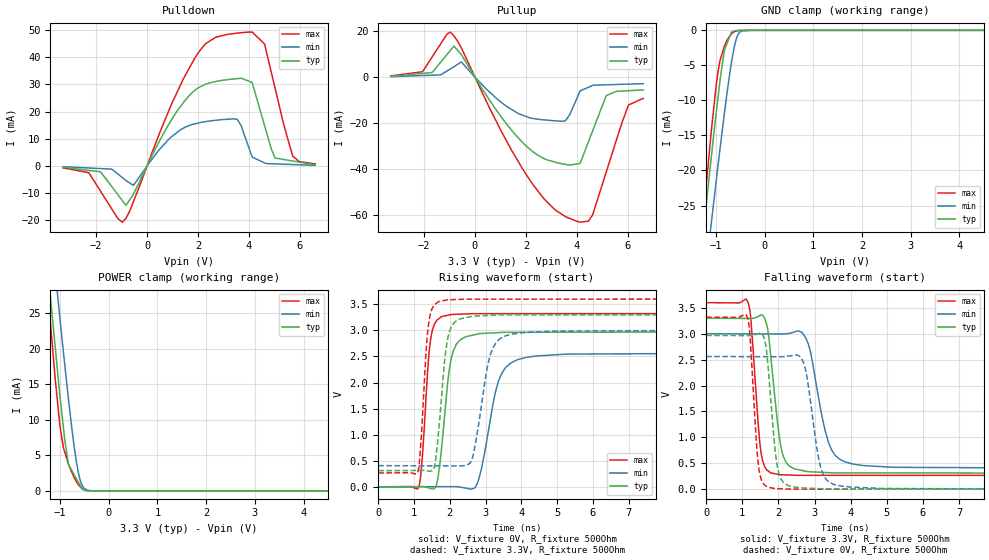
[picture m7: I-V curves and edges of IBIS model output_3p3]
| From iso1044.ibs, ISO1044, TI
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|   output_3p3 Model
[Model]   output_3p3
Model_type   3-state
Polarity   Inverting
Vmeas = 1.65
Vref = 0
Cref = 2pF
Rref = 100000
|   typ   min   max
C_comp   1.207pF   1.163pF   1.293pF
|C_comp_pullup   1.116pF   1.152pF   1.147pF
|C_comp_pulldown   1.051pF   1.086pF   1.093pF
|  Where Nom  PVT is Nominal Process, 3.3V,   27C
|   Fast PVT is Strong Process,  3.0V,   -40C
|   Slow PVT is Weak Process,   3.6V,   150C
[Voltage Range]   3.3   3   3.6
|Junction Temperature
[Temperature Range]   27   150   -40
[Pullup Reference]   3.3   3   3.6
[Pulldown Reference]   0   0   0
[Power Clamp Reference]   3.3   3   3.6
[GND Clamp Reference]   0   0   0
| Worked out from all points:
|   slope of the pulldown table from 0 to 0.495 V, typ, clamps not added: 53.2 ohm
|   slope of the pullup table from 0 to 0.495 V, typ, clamps not added: 56.8 ohm
|   GND clamp passes 1 mA (typ) near -0.72 V on its own axis
|   POWER clamp passes 1 mA (typ) near -0.60 V on its own axis
|   falling waveform, V_fixture 3.3V, R_fixture 500Ohm: 20-80 % time 280ps typ, 442ps min, 206ps max; typ from 3.3 V to 0.31 V
|   rising waveform, V_fixture 0V, R_fixture 500Ohm: 20-80 % time 270ps typ, 441ps min, 192ps max; typ from 0 V to 2.97 V
|   rising waveform, V_fixture 3.3V, R_fixture 500Ohm: 20-80 % time 241ps typ, 373ps min, 177ps max; typ from 0.31 V to 3.3 V
|   falling waveform, V_fixture 0V, R_fixture 500Ohm: 20-80 % time 224ps typ, 322ps min, 175ps max; typ from 2.97 V to 0 V
[Pulldown]
|   Voltage   I(typ)   I(min)   I(max)
-3.3V     -457.3uA   -258uA     -669.3uA
-2.283V   -1.618mA   -733.3uA   -2.463mA
-965.9mV  -12.74mA   -4.286mA   -20.68mA
-542.2mV  -10.56mA   -7.1mA     -13.32mA
871.8mV   15.6mA     10.03mA    20.74mA
2.011V    28.78mA    15.81mA    41.7mA
3.548V    32.16mA    17.07mA    48.91mA
3.983V    31.25mA    7.027mA    49.28mA
4.61V     14.86mA    1.146mA    44.88mA
5.023V    2.931mA    776.7uA    28.62mA
5.712V    1.841mA    543.7uA    3.669mA
6.6V      438.1uA    243.9uA    769.3uA
[GND Clamp]
|   Voltage   I(typ)   I(min)   I(max)
-3.3V     -171.9mA   -168.4mA   -191.9mA
-1.407V   -38.97mA   -46.94mA   -38.27mA
-1.251V   -28.45mA   -37.22mA   -26.03mA
-1.092V   -18mA      -27.4mA    -14.24mA
-951.9mV  -9.366mA   -19.05mA   -5.726mA
-825mV    -2.851mA   -11.84mA   -2.254mA
-683.5mV  -286.5uA   -4.778mA   -529.6uA
-631.5mV  -111.6uA   -2.723mA   -259.4uA
-587.3mV  -58.24uA   -1.392mA   -116.7uA
-514.2mV  -19.13uA   -303uA     -17.74uA
-283.7mV  -378.8nA   -759.8nA   -1.693uA
6.6V      0A         0A         0A
[Pullup]
|   Voltage   I(typ)   I(min)   I(max)
-3.3V     388.9uA    221.3uA    547uA
-2.056V   1.635mA    714.4uA    2.367mA
-965.6mV  11.67mA    3.571mA    19.67mA
-542.2mV  9.963mA    6.597mA    12.92mA
1.04V     -17.49mA   -11.08mA   -23.72mA
2.262V    -32.42mA   -18.02mA   -46.69mA
3.549V    -38.08mA   -19.03mA   -60.86mA
4.125V    -37.64mA   -6.011mA   -63.3mA
4.614V    -23.53mA   -3.633mA   -60.19mA
5.151V    -8.01mA    -3.324mA   -41.38mA
6.024V    -5.917mA   -3.036mA   -12.14mA
6.6V      -5.542mA   -2.845mA   -9.256mA
[POWER Clamp]
|   Voltage   I(typ)   I(min)   I(max)
-3.3V     192.5mA    190.9mA    209.9mA
-1.245V   30.92mA    41.1mA     27.45mA
-1.155V   24.2mA     34.76mA    20.27mA
-1.097V   20.1mA     30.73mA    15.64mA
-1.002V   13.36mA    24.26mA    9.17mA
-931.7mV  8.996mA    19.59mA    6.115mA
-825mV    3.671mA    12.77mA    3.711mA
-666.4mV  1.747mA    4.201mA    1.334mA
-588.1mV  797.4uA    1.544mA    613.3uA
-542.1mV  239.5uA    724.1uA    283.8uA
-229.9mV  7.237uA    1.239uA    35.74nA
6.6V      0A         0A         0A
[Ramp]
R_load = 500
|   typ   min   max
dV/dt_r   1.781/2.69295e-10   1.53606/4.38846e-10   1.99298/1.91584e-10
dV/dt_f   1.79401/2.77586e-10   1.55592/4.40585e-10   2.00061/2.05386e-10
[Falling Waveform]
V_fixture = 3.3V
V_fixture_min = 3V
V_fixture_max = 3.6V
R_fixture = 500Ohm
C_fixture = 0F
|   Time   V(typ)   V(min)   V(max)
0s        3.3V       3V         3.6V
1.155ns   3.296V     2.998V     3.613V
1.512ns   3.361V     2.997V     743.3mV
1.782ns   2.614V     2.996V     318mV
2.08ns    780.9mV    2.996V     278.1mV
2.43ns    394.6mV    3.032V     270.2mV
2.824ns   337.4mV    2.809V     267.4mV
3.381ns   319mV      913.1mV    267.3mV
3.841ns   314.4mV    526.7mV    267.2mV
10ns      310mV      406.6mV    265.6mV
[Rising Waveform]
V_fixture = 0V
V_fixture_min = 0V
V_fixture_max = 0V
R_fixture = 500Ohm
C_fixture = 0F
|   Time   V(typ)   V(min)   V(max)
0s        -629.6nV   139.6uV    -7.043nV
1.136ns   4.129mV    2.108mV    -2.211mV
1.454ns   -28.16mV   2.658mV    2.768V
1.762ns   678.5mV    3.192mV    3.259V
2.04ns    2.453V     3.674mV    3.303V
2.44ns    2.876V     -23.51mV   3.315V
2.824ns   2.936V     176.7mV    3.319V
3.381ns   2.957V     2.06V      3.32V
3.881ns   2.963V     2.433V     3.32V
10ns      2.968V     2.56V      3.322V
[Rising Waveform]
V_fixture = 3.3V
V_fixture_min = 3V
V_fixture_max = 3.6V
R_fixture = 500Ohm
C_fixture = 0F
|   Time   V(typ)   V(min)   V(max)
0s        310mV      406.6mV    265.6mV
1.111ns   313.8mV    403.5mV    291.9mV
1.393ns   303.9mV    402.7mV    3.043V
1.672ns   937.3mV    402mV      3.545V
1.93ns    2.795V     401.2mV    3.586V
2.28ns    3.219V     400.3mV    3.594V
2.637ns   3.27V      558.5mV    3.598V
3.121ns   3.287V     2.497V     3.598V
3.551ns   3.295V     2.893V     3.598V
10ns      3.3V       3V         3.6V
[Falling Waveform]
|Gnd
V_fixture = 0V
V_fixture_min = 0V
V_fixture_max = 0V
R_fixture = 500Ohm
C_fixture = 0F
|   Time   V(typ)   V(min)   V(max)
0s        2.968V     2.56V      3.322V
1.136ns   2.964V     2.558V     3.325V
1.445ns   3V         2.558V     469.5mV
1.692ns   2.537V     2.558V     43.88mV
1.96ns    479.8mV    2.557V     9.597mV
2.25ns    78.28mV    2.567V     3.391mV
2.702ns   22.4mV     2.424V     1.158mV
3.161ns   9.06mV     442.1mV    1.085mV
3.511ns   4.31mV     96.52mV    1.029mV
10ns      -149.8nV   139.7uV    -8.936nV
